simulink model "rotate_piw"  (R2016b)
settings: Solver=ode4  StartTime=0.0  StopTime=trun  FixedStep=step_sz  RelTol=1e-7  EnableMultiTasking=on
PreLoadFcn:
  | env_timeOpt2nd
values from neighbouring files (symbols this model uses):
  A = [0 1;-(w)^2 0;]    [figure_4.m]    (also in figure_3.m; figure_2.m; results.m)
  B = [0; bo]    [figure_4.m]    (also in figure_3.m; figure_2.m; results.m)
  Xo = [8.665 4229]    [figure_4.m]    (also in figure_3.m = [2*c, 0]; figure_2.m = [curves_optx1(k), curves_optx2(k)]; results.m = [3.0*c,0])
libraries: simulink x3

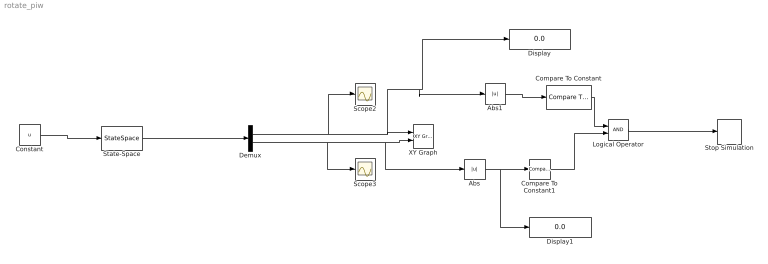
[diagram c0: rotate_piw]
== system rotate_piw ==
  Abs : Abs  Commented=on
  Abs1 : Abs  Commented=on
  Compare To Constant : simulink/Logic and Bit Operations/Compare To Constant  Commented=on  relop=<  const=2.6*10^-9  OutDataTypeStr=boolean
  Compare To Constant1 : simulink/Logic and Bit Operations/Compare To Constant  Commented=on  relop=<=  const=.1  OutDataTypeStr=boolean
  Constant : Constant  Value=u
  Demux : Demux  Outputs=[1, 1]
  Display : Display
  Display1 : Display
  Logical Operator : Logic  Commented=on  AllPortsSameDT=off  OutDataTypeStr=boolean
  Scope2 : Scope
  Scope3 : Scope
  State-Space : StateSpace  A=A  B=B  C=eye(2)  D=[0;0]  X0=Xo  ContinuousStateAttributes="{'xx1',  'xx2'}"
  Stop Simulation : Stop  Commented=on
  XY Graph : simulink/Sinks/XY Graph  Commented=on  xmin=-25  xmax=25  ymin=-20000  ymax=20000  st=-1
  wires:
  Demux/1 -> Scope2/1, Abs1/1, Display/1, XY Graph/1
  Demux/2 -> Scope3/1, Abs/1, XY Graph/2
  State-Space/1 -> Demux/1
  Compare To Constant/1 -> Logical Operator/1
  Logical Operator/1 -> Stop Simulation/1
  Compare To Constant1/1 -> Logical Operator/2
  Abs/1 -> Compare To Constant1/1, Display1/1
  Abs1/1 -> Compare To Constant/1
  Constant/1 -> State-Space/1
